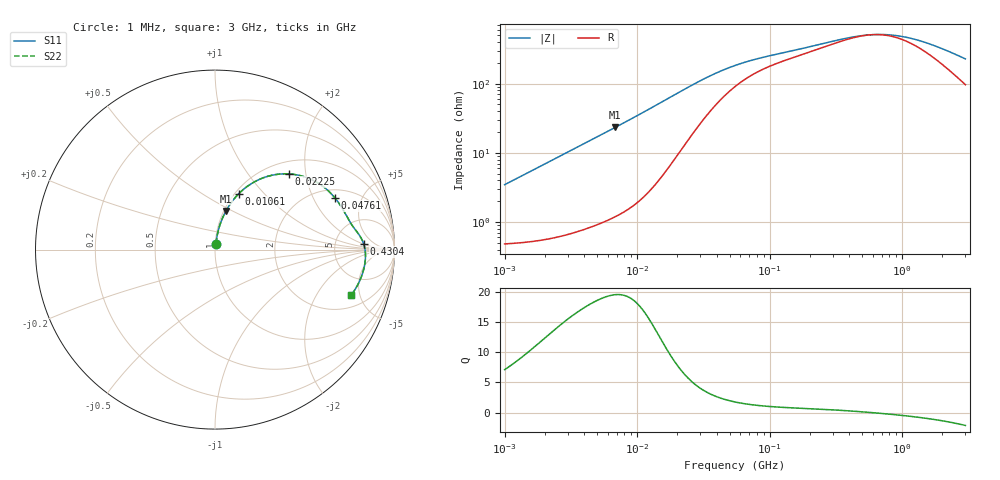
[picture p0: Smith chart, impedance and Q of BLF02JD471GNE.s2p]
! BLF02JD471GNE
# Hz S RI R 50
!Freq.(Hz) S11(Real) S11(Imag) S21(Real) S21(Imag) S12(Real) S12(Imag) S22(Real) S22(Imag)
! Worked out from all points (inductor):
!   401 points, 1 MHz to 3 GHz, reference 50 ohm
!   read as one part in series: L = 546 nH near 1.041 MHz
!   highest Q = 19.5 at 6.831 MHz (marker M1), where L = 542 nH
!   self-resonance near 587.2 MHz
!   S11 on the Smith chart (normalised r, x): 1 MHz: 1.01, +0.07; 10.61 MHz: 1.04, +0.73; 22.25 MHz: 1.24, +1.60; 47.61 MHz: 2.44, +2.99; 430.4 MHz: 10, +2; 3 GHz: 2.94, -4.13
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1000000  0.00596 0.0339  0.994 -0.0339  0.994 -0.0339  0.00596 0.0339
2055611  0.0104 0.0692  0.9896 -0.0692  0.9896 -0.0692  0.0104 0.0692
3823119  0.0239 0.1263  0.9761 -0.1263  0.9761 -0.1263  0.0239 0.1263
6831390  0.0615 0.2159  0.9385 -0.2159  0.9385 -0.2159  0.0615 0.2159
1.061086e7  0.1321 0.3112  0.8679 -0.3112  0.8679 -0.3112  0.1321 0.3112
1.461624e7  0.2271 0.3815  0.7729 -0.3815  0.7729 -0.3815  0.2271 0.3815
1.821614e7  0.3173 0.4142  0.6827 -0.4142  0.6827 -0.4142  0.3173 0.4142
2.225279e7  0.4095 0.4218  0.5905 -0.4218  0.5905 -0.4218  0.4095 0.4218
2.664524e7  0.491 0.4078  0.509 -0.4078  0.509 -0.4078  0.491 0.4078
3.320783e7  0.5761 0.3695  0.4239 -0.3695  0.4239 -0.3695  0.5761 0.3695
3.976269e7  0.6293 0.3292  0.3707 -0.3292  0.3707 -0.3292  0.6293 0.3292
4.761141e7  0.6684 0.288  0.3316 -0.288  0.3316 -0.288  0.6684 0.288
5.477226e7  0.6909 0.2581  0.3091 -0.2581  0.3091 -0.2581  0.6909 0.2581
9.593103e7  0.7436 0.1685  0.2564 -0.1685  0.2564 -0.1685  0.7436 0.1685
2.094008e8  0.7924 0.0971  0.2076 -0.0971  0.2076 -0.0971  0.7924 0.0971
4.304467e8  0.8283 0.0321  0.1717 -0.0321  0.1717 -0.0321  0.8283 0.0321
5.929311e8  0.8361 -0.00106  0.1639 0.00106  0.1639 0.00106  0.8361 -0.00106
8.005644e8  0.8385 -0.0349  0.1615 0.0349  0.1615 0.0349  0.8385 -0.0349
1.038491e9  0.8364 -0.0674  0.1636 0.0674  0.1636 0.0674  0.8364 -0.0674
1.374365e9  0.8292 -0.1072  0.1708 0.1072  0.1708 0.1072  0.8292 -0.1072
2.050964e9  0.8054 -0.1756  0.1946 0.1756  0.1946 0.1756  0.8054 -0.1756
3e9  0.7583 -0.2538  0.2417 0.2538  0.2417 0.2538  0.7583 -0.2538
